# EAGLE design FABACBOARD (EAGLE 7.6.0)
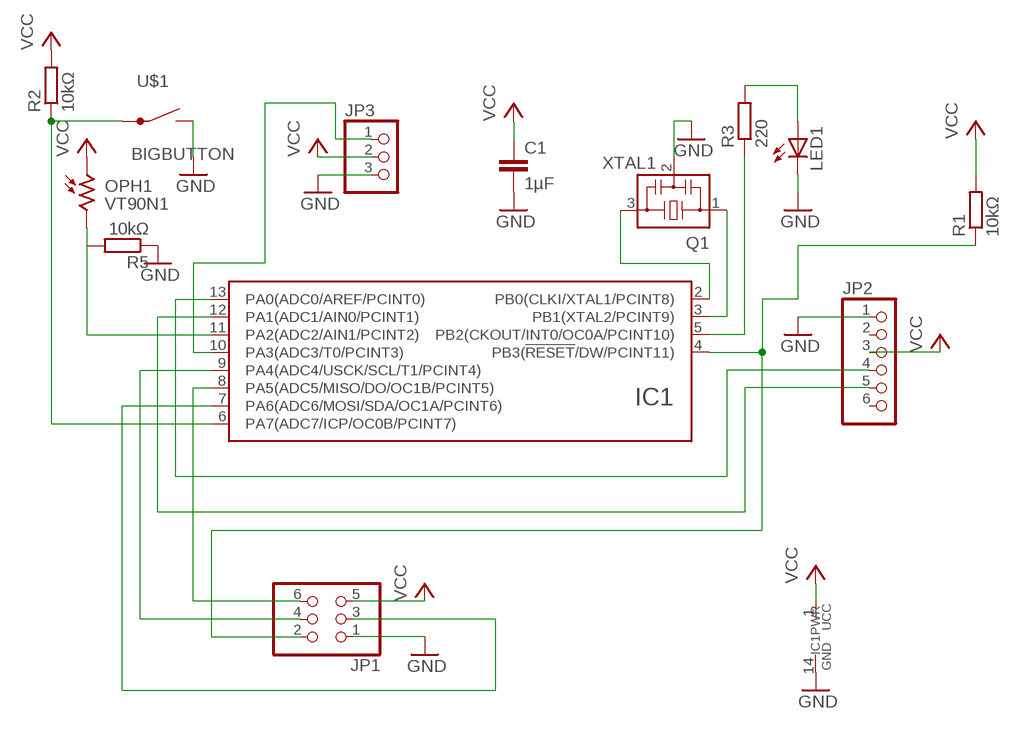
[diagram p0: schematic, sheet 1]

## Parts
C1  1µF  C-EUC1206  [C1206]
IC1  ATTINY24/44/84-SSU  [SOIC14]
JP1  PINHD-2X3  [2X03]
JP2  PINHD-1X6  [1X06]
JP3  PINHD-1X3  [1X03]
LED1  LEDCHIPLED_1206  [CHIPLED_1206]
OPH1  VT90N1  [VT900]
Q1  XTAL1  CSTCR6M00G53Z  [CSTCR6M]
R1  10kΩ  R-EU_M1206  [M1206]
R2  10kΩ  R-EU_M1206  [M1206]
R3  220  R-EU_M1206  [M1206]
R5  10kΩ  R-EU_M1206  [M1206]
U$1  BIGBUTTON  [BIGBUTTON]

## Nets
GND: C1.2 IC1.14(GND) JP1.1 JP2.1 JP3.3 LED1.C Q1.2 R5.1 U$1.2A U$1.2B(2A)
N$1: IC1.2(PB0(CLKI/XTAL1/PCINT8)) Q1.3
N$2: IC1.3(PB1(XTAL2/PCINT9)) Q1.1
N$3: IC1.7(PA6(ADC6/MOSI/SDA/OC1A/PCINT6)) JP1.3
N$4: IC1.13(PA0(ADC0/AREF/PCINT0)) JP2.4
N$5: IC1.12(PA1(ADC1/AIN0/PCINT1)) JP2.5
N$6: IC1.8(PA5(ADC5/MISO/DO/OC1B/PCINT5)) JP1.6
N$7: IC1.9(PA4(ADC4/USCK/SCL/T1/PCINT4)) JP1.4
N$8: IC1.4(PB3(!RESET!/DW/PCINT11)) JP1.2 R1.1
N$9: IC1.6(PA7(ADC7/ICP/OC0B/PCINT7)) R2.1 U$1.1A U$1.1B(1A)
N$10: LED1.A R3.2
N$11: IC1.5(PB2(CKOUT/INT0/OC0A/PCINT10)) R3.1
N$12: IC1.11(PA2(ADC2/AIN1/PCINT2)) OPH1.2 R5.2
N$13: IC1.10(PA3(ADC3/T0/PCINT3)) JP3.1
VCC: C1.1 IC1.1(UCC) JP1.5 JP2.3 JP3.2 OPH1.1 R1.2 R2.2
Unconnected: JP2.2 JP2.6

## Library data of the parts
C1 = rcl:C-EU: CAPACITOR, European symbol
IC1 = atmel_tiny24-44-84tiny48-88mega48-88-168-328:ATTINY24/44/84
JP1 = pinhead:PINHD-2X3: PIN HEADER
JP2 = pinhead:PINHD-1X6: PIN HEADER
JP3 = pinhead:PINHD-1X3: PIN HEADER
LED1 = led:LED: LED
OPH1 = photo-elements:VT9: Photoconductive Cell VT900 Series
Q1 = murata-filter:CSTCR: Resonator Source: murata.co.jp; MPN: CSTCR6M00G53-R0; OC_FARNELL: 1170434; OC_NEWARK: 25M8759
R1-R3 R5 = rcl:R-EU_: RESISTOR, European symbol
U$1 = LAHAYELIB:BIGBUTTON

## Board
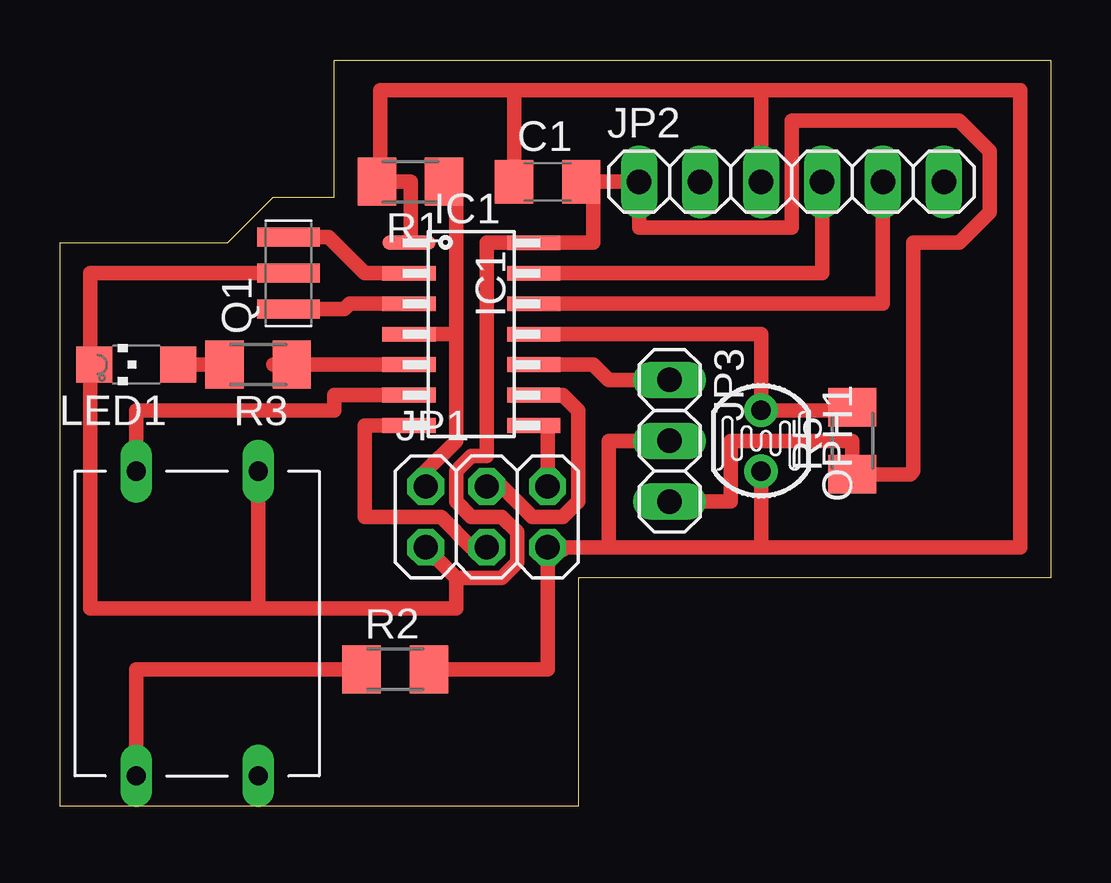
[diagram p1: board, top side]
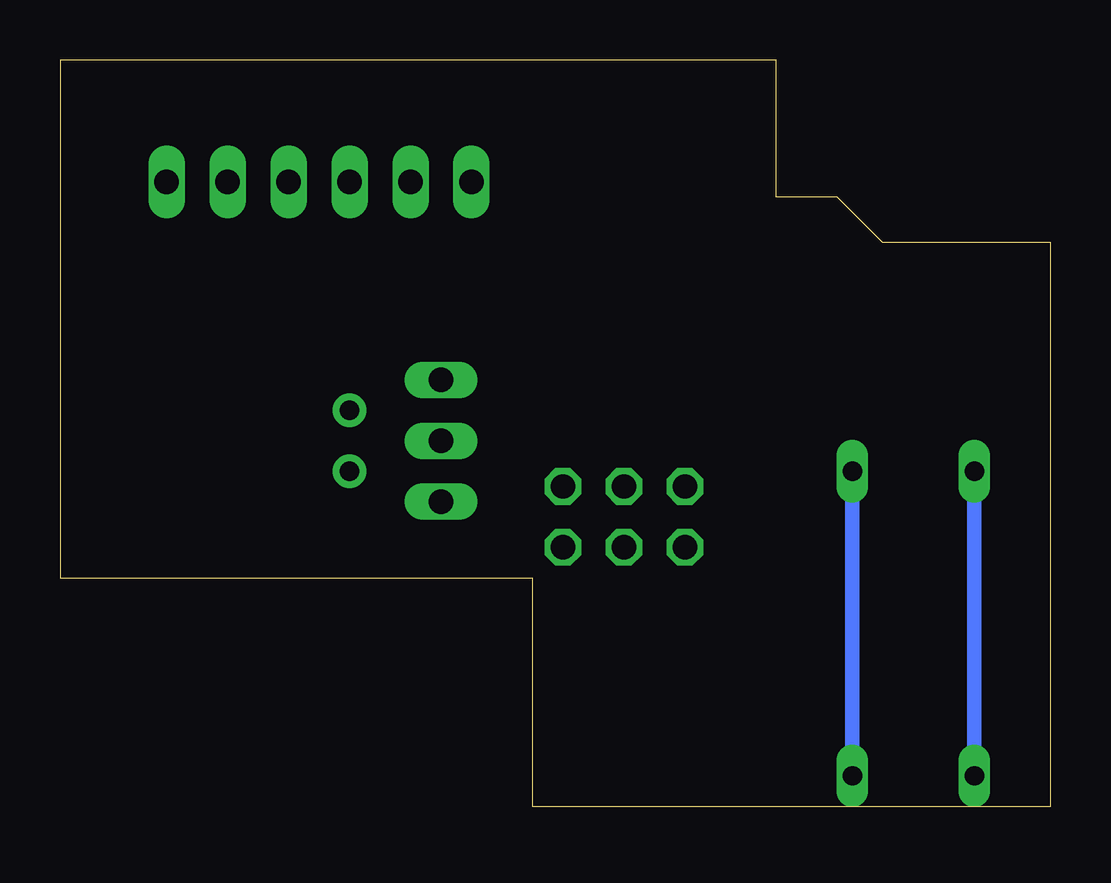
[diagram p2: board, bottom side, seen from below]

Size 41.28 x 31.11 mm. Coordinates in mm from the lower left corner, seen from the top.
Outline: 0,23.5 6.99,23.5 8.89,25.4 11.43,25.4 11.43,31.11 41.28,31.11 41.28,9.53 21.59,9.53 21.59,0 0,0 0,23.5
Copper layers (1*16): Top 0.035mm / dielectric 1.5mm / Bottom 0.035mm
Design rules "default": minimum track width 10mil, minimum drill 24mil, track to track 8mil, track to pad 8mil, pad to pad 8mil, via to via 8mil, smd to smd 8mil, copper to edge 40mil, drill to drill 8mil, minimum pad ring 10mil, minimum via ring 8mil, stop-mask expansion 4mil, vias tented up to drill 0mil, thermal gap 10mil

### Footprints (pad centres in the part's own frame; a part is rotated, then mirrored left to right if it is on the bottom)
C1206 = smd 1.6 x 1.8: 1 -1.4,0; 2 1.4,0
SOIC14 = smd 0.61 x 2.21: 1 -3.81,-2.603; 2 -2.54,-2.603; 3 -1.27,-2.603; 4 0,-2.603; 5 1.27,-2.603; 6 2.54,-2.603; 7 3.81,-2.603; 8 3.81,2.603; 9 2.54,2.603; 10 1.27,2.603; 11 0,2.603; 12 -1.27,2.603; 13 -2.54,2.603; 14 -3.81,2.603
2X03 = drill 1.016 octagon: 1 -2.54,-1.27; 2 -2.54,1.27; 3 0,-1.27; 4 0,1.27; 5 2.54,-1.27; 6 2.54,1.27
1X06 = drill 1.016 long: 1 -6.35,0; 2 -3.81,0; 3 -1.27,0; 4 1.27,0; 5 3.81,0; 6 6.35,0
1X03 = drill 1.016 long: 1 -2.54,0; 2 0,0; 3 2.54,0
CHIPLED_1206 = smd 1.5 x 1.5: A 0,-1.75; C 0,1.75
VT900 = drill 0.8 pad 1.4: 1 -1.27,0; 2 1.27,0
CSTCR6M = smd 0.8 x 2.6: 1 -1.5,0; 2 0,0; 3 1.5,0
M1206 = smd 1.6 x 2: 1 -1.4,0; 2 1.4,0
BIGBUTTON = drill 0.8 long: 1A -7.62,2.54; 1B 5.08,2.54; 2A -7.62,-2.54; 2B 5.08,-2.54

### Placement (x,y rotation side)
C1  20.32,26.04 0 top
IC1  17.14,19.68 270 top
JP1  17.78,12.07 0 top
JP2  30.48,26.04 0 top
JP3  25.4,15.24 270 top
LED1  3.18,18.42 90 top
OPH1  29.21,15.24 90 top
Q1  9.53,22.22 90 top
R1  14.61,26.04 180 top
R2  13.97,5.71 0 top
R3  8.26,18.42 180 top
R5  33.02,15.24 90 top
U$1  5.71,8.89 90 top

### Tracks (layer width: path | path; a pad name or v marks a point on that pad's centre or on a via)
GND
  Top 0.61: 16.51,9.53 18.42,9.53 19.05,10.16 19.05,11.43 18.42,12.07 17.14,12.07 16.51,12.7 16.51,13.97 17.14,14.61 17.78,14.61 17.78,23.5 IC1.14 22.22,23.5 22.22,26.04 C1.2 JP2.1 24.13,24.13 30.48,24.13 30.48,28.57 37.47,28.57 38.73,27.31 38.73,24.76 37.47,23.5 35.56,23.5 35.56,13.97 35.43,13.84 R5.1 33.02,15.24 27.94,15.24 27.94,12.7 JP3.3 | 16.51,9.53 JP1.1 | Q1.2 1.27,22.22 1.27,18.42 | 16.51,9.53 16.51,8.25 8.26,8.25 | U$1.2B 8.26,8.25 | LED1.C 1.27,18.42 | 8.26,8.25 1.27,8.25 1.27,18.42
  Bottom 0.61: U$1.2A U$1.2B
N$1
  Top 0.61: Q1.3 11.2,23.72 12.7,22.22 IC1.2
N$2
  Top 0.61: Q1.1 11.84,20.72 12.07,20.96 IC1.3
N$3
  Top 0.61: JP1.3 17.14,10.79 15.88,12.07 12.7,12.07 12.7,15.87 IC1.7
N$4
  Top 0.61: IC1.13 31.75,22.22 JP2.4
N$5
  Top 0.61: IC1.12 34.29,20.96 JP2.5
N$6
  Top 0.61: IC1.8 20.32,15.87 JP1.6
N$7
  Top 0.61: IC1.9 20.96,17.14 21.59,16.51 21.59,12.7 20.96,12.07 19.68,12.07 18.42,13.33 JP1.4
N$8
  Top 0.61: 16.51,19.68 16.51,15.24 15.24,13.97 JP1.2 | 16.51,19.68 16.51,26.54 | IC1.4 16.51,19.68 | 16.51,26.67 16.51,26.54 | 16.51,26.54 R1.1
N$9
  Top 0.61: IC1.6 11.43,17.14 11.43,16.51 3.18,16.51 U$1.1B | U$1.1A 3.18,5.71 R2.1
  Bottom 0.61: U$1.1B U$1.1A
N$10
  Top 0.61: LED1.A R3.2
N$11
  Top 0.61: IC1.5 R3.1 8.89,18.42
N$12
  Top 0.61: IC1.11 29.21,19.68 OPH1.2 32.89,16.51 R5.2
N$13
  Top 0.61: JP3.1 22.86,17.78 22.22,18.42 IC1.10
VCC
  Top 0.61: IC1.1 14.61,23.5 14.61,26.04 13.34,26.04 | R1.2 13.34,26.04 | 13.34,26.04 13.34,29.85 18.92,29.85 | 18.92,29.85 C1.1 | 18.92,29.85 29.21,29.85 | JP2.3 29.21,29.85 | 29.21,29.85 40,29.85 40,10.79 29.21,10.79 | R2.2 20.32,5.71 JP1.5 | 20.96,10.7 JP1.5 | 29.21,10.79 OPH1.1 | 29.21,10.79 22.86,10.79 | 22.86,10.79 JP1.5 | JP3.2 22.86,15.24 22.86,10.79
